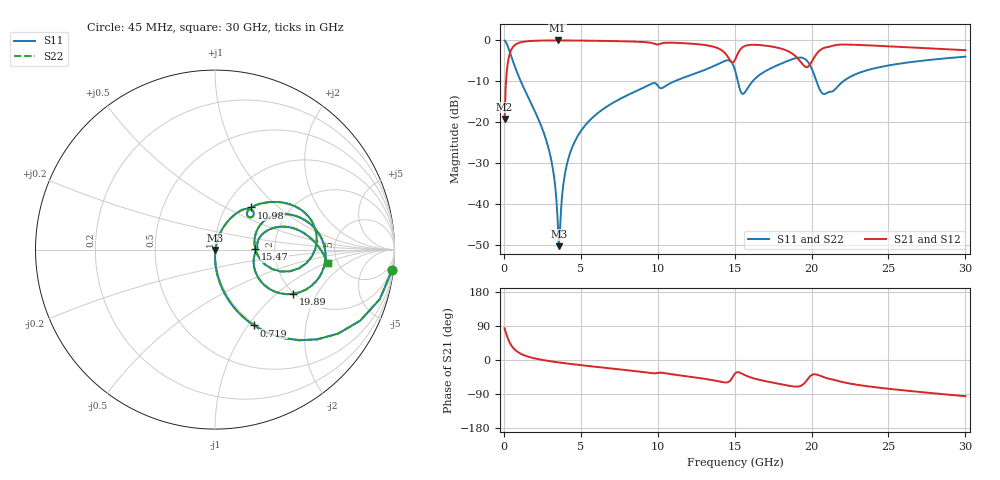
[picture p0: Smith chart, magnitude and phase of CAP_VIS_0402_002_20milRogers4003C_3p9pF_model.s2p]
! S-parameter model data by Modelithics Inc.  support@modelithics.com  813-866-6335  Tampa FL USA
! S-Parameter data specifications:
! Substrate: 20-mil Rogers 4003C, substrate thickness, H=0.508mm, Dielectric constant, Er=3.75
! PCB Mounting Pad Footprint: Pad width, PadW=0.50mm , Pad length, PadL=0.50mm , Pad gap, PadG (edge-to-edge)=0.40mm , Reference planes=1.4mm apart
! Created Wed Nov 18 12:47:06 2015
# hz S ma R 50
! 2 Port Network Data from SP1.SP block
! freq  magS11  angS11  magS21  angS21  magS12  angS12  magS22  angS22
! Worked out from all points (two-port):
!   401 points, 45 MHz to 30 GHz, reference 50 ohm
!   highest |S21| = -0.03 dB at 3.49 GHz (marker M1); lowest = -19.1 dB at 45 MHz (marker M2)
!   |S21| within 3 dB of the highest: 401.4 MHz to 14.35 GHz (13.95 GHz wide, 189 % of centre); 20.38 GHz to end of sweep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
!   lowest |S11| = -50.2 dB at 3.565 GHz (marker M3), VSWR 1.01, Z = 50.3 - j0.147 ohm
!   |S11| at or under -10 dB: 1.099 GHz to 11.07 GHz (9.976 GHz wide, 164 % of centre); 15.21 GHz to 16.16 GHz (956.3 MHz wide, 6.1 % of centre); 20.32 GHz to 22.05 GHz (1.731 GHz wide, 8.17 % of centre)
!   |S22| runs from -50.2 to -0.1 dB; largest |S21 - S12| = 0
!   S11 on the Smith chart (normalised r, x): 45 MHz: 1, -18; 719 MHz: 0.98, -1.07; 10.98 GHz: 1.31, +0.68; 15.47 GHz: 1.58, +0.01; 19.89 GHz: 1.98, -1.31; 30 GHz: 4.16, -1.06
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4.5e7  0.9939 -6.4  0.1105 83.6  0.1105 83.6  0.9939 -6.4
3.4455e8  0.7581 -41.3  0.6515 48.7  0.6515 48.7  0.7581 -41.3
7.189875e8  0.4749 -62.8  0.8788 27.0  0.8788 27.0  0.4749 -62.8
2.815838e9  0.05521 -89.3  0.9958 -2.0  0.9958 -2.0  0.05521 -89.3
3.190275e9  0.0266 -88.4  0.9968 -4.3  0.9968 -4.3  0.0266 -88.4
3.489825e9  0.006635 -70.6  0.997 -6.0  0.997 -6.0  0.006635 -70.6
3.564712e9  0.003102 -28.2  0.997 -6.4  0.997 -6.4  0.003102 -28.2
4.163812e9  0.03471 75.3  0.9961 -9.6  0.9961 -9.6  0.03471 75.3
5.062462e9  0.08138 73.6  0.993 -13.9  0.993 -13.9  0.08138 73.6
1.007992e10  0.2692 41.8  0.8968 -33.5  0.8968 -33.5  0.2692 41.8
1.097858e10  0.3103 49.2  0.9357 -38.1  0.9357 -38.1  0.3103 49.2
1.389919e10  0.5114 27.7  0.8038 -55.9  0.8038 -55.9  0.5114 27.7
1.464806e10  0.5685 4.6  0.5924 -56.6  0.5924 -56.6  0.5685 4.6
1.50225e10  0.434 -16.2  0.58 -35.8  0.58 -35.8  0.434 -16.2
1.547182e10  0.2242 1.1  0.8115 -36.0  0.8115 -36.0  0.2242 1.1
1.786822e10  0.5056 20.7  0.8072 -62.9  0.8072 -62.9  0.5056 20.7
1.92162e10  0.6171 -4.1  0.5692 -69.3  0.5692 -69.3  0.6171 -4.1
1.989019e10  0.5018 -29.4  0.5052 -43.5  0.5052 -43.5  0.5018 -29.4
2.003996e10  0.4386 -33.8  0.5618 -39.1  0.5618 -39.1  0.4386 -33.8
2.086372e10  0.2222 -7.9  0.8155 -46.2  0.8155 -46.2  0.2222 -7.9
2.505742e10  0.4966 11.3  0.8449 -76.1  0.8449 -76.1  0.4966 11.3
3e10  0.6329 -6.9  0.7585 -95.6  0.7585 -95.6  0.6329 -6.9
